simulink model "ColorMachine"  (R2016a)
settings: Solver=FixedStepAuto  StartTime=0.0  StopTime=inf  RelTol=1e-3
libraries: miniQ x2

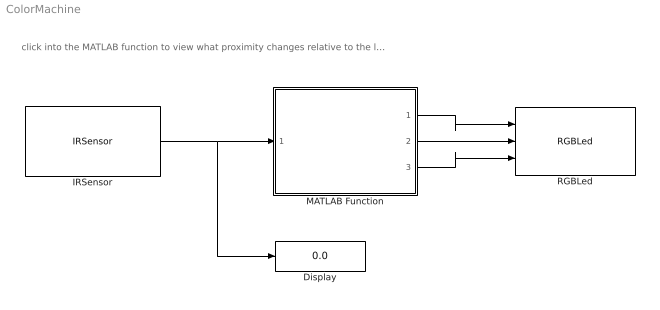
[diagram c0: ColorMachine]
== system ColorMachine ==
  note: click into the MATLAB function to view what proximity changes relative to the light color
  Display : Display
  IRSensor : miniQ/IRSensor  sampleTime_dd=0.01  debug_dd=off
  MATLAB Function : MATLAB Function  TreatAsAtomicUnit=on
  RGBLed : miniQ/RGBLed
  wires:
  IRSensor/1 -> Display/1, MATLAB Function/1(proximity)
  MATLAB Function/1(red) -> RGBLed/1
  MATLAB Function/2(green) -> RGBLed/2
  MATLAB Function/3(blue) -> RGBLed/3

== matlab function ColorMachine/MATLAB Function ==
function [red,green,blue] = colormachine(proximity)
if proximity <5
    red = 0;
    green=255;
    blue = 0;
elseif proximity>5&&proximity<30 
    red = 0;
    green=0;
    blue = 255;
else
   red = 255;
   green=0;
   blue = 0;  
    
end
